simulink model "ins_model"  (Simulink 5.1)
settings: Solver=ode45  StartTime=0.0  StopTime=max(Time__s_)  RelTol=1e-3
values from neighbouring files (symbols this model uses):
  hid = [-0.2304    0.7148   -0.6309   -0.0280    0.1870    0.0308   -0.0329   -0.0106]    [meen.m]
  hir = [-0.0106   -0.0329    0.0308    0.1870   -0.0280   -0.6309    0.7148   -0.2304]    [meen.m]
  K = eye(3)    [meen.m]
  lod = [-0.0106    0.0329    0.0308  -0.1870   -0.0280    0.6309    0.7148    0.2304]    [meen.m]
  lor = [0.2304    0.7148    0.6309   -0.0280   -0.1870    0.0308    0.0329   -0.0106]    [meen.m]
  xaccel = X_Accel__g_ - mean(X_Accel__g_)    [meen.m]
  yaccel = Y_Accel__g_ - mean(Y_Accel__g_)    [meen.m]
  zaccel = Z_Accel__g_ - mean(Z_Accel__g_)    [meen.m]
undefined symbols (not defined in the file or in its folder): Customize, dspblkfdatool, Pitch__deg_, Roll__deg_, X_Accel__g_, Y_Accel__g_, Yaw_rate__deg_s_, Z_Accel__g_
libraries: dspmlti3 x12, dspsigattribs x9, simulink x3, simulink_extras x1

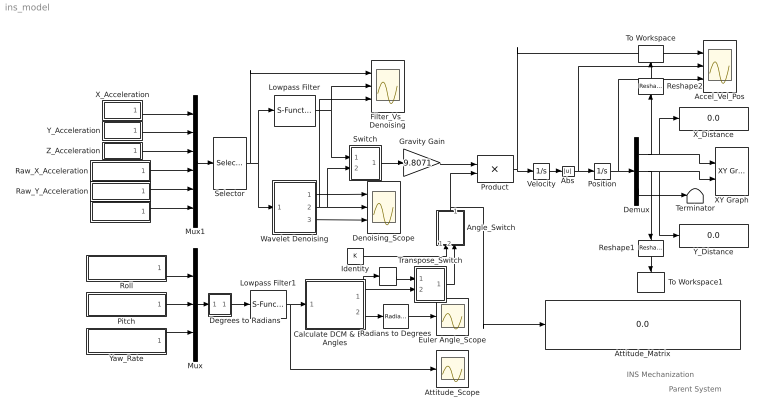
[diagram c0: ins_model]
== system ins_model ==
  note: INS Mechanization
  note: Parent System
  "    " : S-Function  FunctionName=sdspmtrnsp2  Parameters=Hermitian  mask(Transpose){Hermitian=off}
      mask help: Compute the matrix transpose. Vector input signals are treated as [Mx1] matrices. The output is always a matrix.
      mask init:
      | if(Hermitian==1),  str = 'u^H';
      | else               str = 'u^T';
      | end
  "               " : Subsystem  mask(Signal From Workspace){X=Z_Accel__g_, Ts=1/132, nsamps=1, OutputAfterFinalValue=Setting to zero}
      mask prompts: X "Signal:"; Ts "Sample time:"; nsamps "Samples per frame:"; OutputAfterFinalValue "Form output after final data value by:"
      mask help: Output signal samples obtained from the MATLAB workspace at successive sample times. A signal matrix is interpreted as having one channel per column. Signal columns may be buffered into frames by specifying a number of samples per frame greater than 1. An M x N x P signal array outputs M x N matrices at successive sample times. The samples per frame must be equal to 1 for 3 dimensional signal arrays.
      mask init:
      | [s,Ts] = dspblksfw2('init', X,Ts,nsamps);
  Abs : Abs
  Accel_Vel_Pos : Scope  NumInputPorts=3
  Angle_Switch : Subsystem  Orientation=up  mask(Manual Switch){sw=0, action=0}
      mask prompts: sw "Current setting:"
      mask help: Output toggles between two inputs by double-clicking on the block.
      mask init:
      | [x,y]=manswitch;
  Attitude_Matrix : Display
  Attitude_Scope : Scope
  Calculate DCM & Euler Angles : Subsystem
  Degrees to Radians : Subsystem
  Demux : Demux  Outputs=3
  Denoising_Scope : Scope  NumInputPorts=3
  Euler Angle_Scope : Scope
  Filter_Vs_Denoising : Scope  NumInputPorts=3
  Gravity Gain : Gain  Gain=9.8071
  Identity : Constant  Value=K
  Lowpass Filter : S-Function  StartFcn=dspblkfdatool('StartFcn');  FunctionName=sdspfilter  Parameters=1, 0, 5, 0, 1, [-0.0021051330842123276, -0.010808692912682402, -0.027404006620206183, -0.040945792508837571, -0.02656378035569611, 0.037365730644418289, 0.14346167047042629, 0.24652272003377734, 0.28957728654925807, 0.24652272003377734, 0.14346167047042629, 0.037365730644418289, -0.02656378035569611, -0.040945792508837571, -0.027404006620206183, -0.010808692912682402, -0.0021051330842123276], [1],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
  Lowpass Filter1 : S-Function  StartFcn=dspblkfdatool('StartFcn');  FunctionName=sdspfilter  Parameters=1, 0, 5, 0, 1, [-0.0021051330842123276, -0.010808692912682402, -0.027404006620206183, -0.040945792508837571, -0.02656378035569611, 0.037365730644418289, 0.14346167047042629, 0.24652272003377734, 0.28957728654925807, 0.24652272003377734, 0.14346167047042629, 0.037365730644418289, -0.02656378035569611, -0.040945792508837571, -0.027404006620206183, -0.010808692912682402, -0.0021051330842123276], [1],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
  Mux : Mux  Inputs=3
  Mux1 : Mux  Inputs=6
  Pitch : Subsystem  mask(Signal From Workspace){X=Pitch__deg_, Ts=1/132, nsamps=1, OutputAfterFinalValue=Setting to zero}
      mask prompts: X "Signal:"; Ts "Sample time:"; nsamps "Samples per frame:"; OutputAfterFinalValue "Form output after final data value by:"
      mask help: Output signal samples obtained from the MATLAB workspace at successive sample times. A signal matrix is interpreted as having one channel per column. Signal columns may be buffered into frames by specifying a number of samples per frame greater than 1. An M x N x P signal array outputs M x N matrices at successive sample times. The samples per frame must be equal to 1 for 3 dimensional signal arrays.
      mask init:
      | [s,Ts] = dspblksfw2('init', X,Ts,nsamps);
  Position : Integrator
  Product : Product  Multiplication=Matrix(*)
  Radians to Degrees : simulink_extras/Transformations/Radians to Degrees
  Raw_X_Acceleration : Subsystem  mask(Signal From Workspace){X=X_Accel__g_, Ts=1/132, nsamps=1, OutputAfterFinalValue=Setting to zero}
      mask prompts: X "Signal:"; Ts "Sample time:"; nsamps "Samples per frame:"; OutputAfterFinalValue "Form output after final data value by:"
      mask help: Output signal samples obtained from the MATLAB workspace at successive sample times. A signal matrix is interpreted as having one channel per column. Signal columns may be buffered into frames by specifying a number of samples per frame greater than 1. An M x N x P signal array outputs M x N matrices at successive sample times. The samples per frame must be equal to 1 for 3 dimensional signal arrays.
      mask init:
      | [s,Ts] = dspblksfw2('init', X,Ts,nsamps);
  Raw_Y_Acceleration : Subsystem  mask(Signal From Workspace){X=Y_Accel__g_, Ts=1/132, nsamps=1, OutputAfterFinalValue=Setting to zero}
      mask prompts: X "Signal:"; Ts "Sample time:"; nsamps "Samples per frame:"; OutputAfterFinalValue "Form output after final data value by:"
      mask help: Output signal samples obtained from the MATLAB workspace at successive sample times. A signal matrix is interpreted as having one channel per column. Signal columns may be buffered into frames by specifying a number of samples per frame greater than 1. An M x N x P signal array outputs M x N matrices at successive sample times. The samples per frame must be equal to 1 for 3 dimensional signal arrays.
      mask init:
      | [s,Ts] = dspblksfw2('init', X,Ts,nsamps);
  Reshape1 : simulink/Math Operations/Reshape  Orientation=down  OutputDimensionality=1-D array  OutputDimensions=[1,1]
  Reshape2 : simulink/Math Operations/Reshape  Orientation=up  OutputDimensionality=1-D array  OutputDimensions=[1,1]
  Roll : Subsystem  mask(Signal From Workspace){X=Roll__deg_, Ts=1/132, nsamps=1, OutputAfterFinalValue=Setting to zero}
      mask prompts: X "Signal:"; Ts "Sample time:"; nsamps "Samples per frame:"; OutputAfterFinalValue "Form output after final data value by:"
      mask help: Output signal samples obtained from the MATLAB workspace at successive sample times. A signal matrix is interpreted as having one channel per column. Signal columns may be buffered into frames by specifying a number of samples per frame greater than 1. An M x N x P signal array outputs M x N matrices at successive sample times. The samples per frame must be equal to 1 for 3 dimensional signal arrays.
      mask init:
      | [s,Ts] = dspblksfw2('init', X,Ts,nsamps);
  Selector : Selector  Elements=[1 2 3]  InputPortWidth=6
  Switch : Subsystem  mask(Manual Switch){sw=0, action=0}
      mask prompts: sw "Current setting:"
      mask help: Output toggles between two inputs by double-clicking on the block.
      mask init:
      | [x,y]=manswitch;
  Terminator : Terminator
  To Workspace : ToWorkspace  VariableName=xout  SampleTime=-1  SaveFormat=Array
  To Workspace1 : ToWorkspace  VariableName=yout  SampleTime=-1  SaveFormat=Array
  Transpose_Switch : Subsystem  mask(Manual Switch){sw=1, action=0}
      mask prompts: sw "Current setting:"
      mask help: Output toggles between two inputs by double-clicking on the block.
      mask init:
      | [x,y]=manswitch;
  Velocity : Integrator
  Wavelet Denoising : Subsystem
  XY Graph : simulink/Sinks/XY Graph  xmin=-300  xmax=300  ymin=-300  ymax=300  st=-1
  X_Acceleration : Subsystem  mask(Signal From Workspace){X=xaccel, Ts=1/132, nsamps=1, OutputAfterFinalValue=Setting to zero}
      mask prompts: X "Signal:"; Ts "Sample time:"; nsamps "Samples per frame:"; OutputAfterFinalValue "Form output after final data value by:"
      mask help: Output signal samples obtained from the MATLAB workspace at successive sample times. A signal matrix is interpreted as having one channel per column. Signal columns may be buffered into frames by specifying a number of samples per frame greater than 1. An M x N x P signal array outputs M x N matrices at successive sample times. The samples per frame must be equal to 1 for 3 dimensional signal arrays.
      mask init:
      | [s,Ts] = dspblksfw2('init', X,Ts,nsamps);
  X_Distance : Display
  Y_Acceleration : Subsystem  mask(Signal From Workspace){X=yaccel, Ts=1/132, nsamps=1, OutputAfterFinalValue=Setting to zero}
      mask prompts: X "Signal:"; Ts "Sample time:"; nsamps "Samples per frame:"; OutputAfterFinalValue "Form output after final data value by:"
      mask help: Output signal samples obtained from the MATLAB workspace at successive sample times. A signal matrix is interpreted as having one channel per column. Signal columns may be buffered into frames by specifying a number of samples per frame greater than 1. An M x N x P signal array outputs M x N matrices at successive sample times. The samples per frame must be equal to 1 for 3 dimensional signal arrays.
      mask init:
      | [s,Ts] = dspblksfw2('init', X,Ts,nsamps);
  Y_Distance : Display
  Yaw_Rate : Subsystem  mask(Signal From Workspace){X=Yaw_rate__deg_s_, Ts=1/132, nsamps=1, OutputAfterFinalValue=Setting to zero}
      mask prompts: X "Signal:"; Ts "Sample time:"; nsamps "Samples per frame:"; OutputAfterFinalValue "Form output after final data value by:"
      mask help: Output signal samples obtained from the MATLAB workspace at successive sample times. A signal matrix is interpreted as having one channel per column. Signal columns may be buffered into frames by specifying a number of samples per frame greater than 1. An M x N x P signal array outputs M x N matrices at successive sample times. The samples per frame must be equal to 1 for 3 dimensional signal arrays.
      mask init:
      | [s,Ts] = dspblksfw2('init', X,Ts,nsamps);
  Z_Acceleration : Subsystem  mask(Signal From Workspace){X=zaccel, Ts=1/132, nsamps=1, OutputAfterFinalValue=Setting to zero}
      mask prompts: X "Signal:"; Ts "Sample time:"; nsamps "Samples per frame:"; OutputAfterFinalValue "Form output after final data value by:"
      mask help: Output signal samples obtained from the MATLAB workspace at successive sample times. A signal matrix is interpreted as having one channel per column. Signal columns may be buffered into frames by specifying a number of samples per frame greater than 1. An M x N x P signal array outputs M x N matrices at successive sample times. The samples per frame must be equal to 1 for 3 dimensional signal arrays.
      mask init:
      | [s,Ts] = dspblksfw2('init', X,Ts,nsamps);
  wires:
  Mux/1 -> Degrees to Radians/1(Degrees in)
  Roll/1(Outport) -> Mux/1
  Pitch/1(Outport) -> Mux/2
  X_Acceleration/1(Outport) -> Mux1/1
  Y_Acceleration/1(Outport) -> Mux1/2
  Z_Acceleration/1(Outport) -> Mux1/3
  Mux1/1 -> Selector/1
  Calculate DCM & Euler Angles/2(Euler) -> Radians to Degrees/1
  Velocity/1 -> Abs/1
  Position/1 -> Demux/1, Accel_Vel_Pos/3
  Demux/1 -> X_Distance/1, XY Graph/1, Reshape2/1
  Demux/2 -> Y_Distance/1, XY Graph/2, Reshape1/1
  Demux/3 -> Terminator/1
  Gravity Gain/1 -> Product/1
  Product/1 -> Velocity/1, Accel_Vel_Pos/1
  Yaw_Rate/1(Outport) -> Mux/3
  Degrees to Radians/1(Radians out) -> Lowpass Filter1/1
  Switch/1(Out1) -> Gravity Gain/1
  Lowpass Filter/1 -> Switch/1(1), Filter_Vs_Denoising/2
  "               "/1(Outport) -> Mux1/6
  Raw_Y_Acceleration/1(Outport) -> Mux1/5
  Raw_X_Acceleration/1(Outport) -> Mux1/4
  Selector/1 -> Lowpass Filter/1, Wavelet Denoising/1(In1), Filter_Vs_Denoising/1
  Radians to Degrees/1 -> Euler Angle_Scope/1
  Angle_Switch/1(Out1) -> Attitude_Matrix/1, Product/2
  Identity/1 -> Angle_Switch/1(1)
  Calculate DCM & Euler Angles/1(DCM) -> Transpose_Switch/2(2), "    "/1
  "    "/1 -> Transpose_Switch/1(1)
  Lowpass Filter1/1 -> Calculate DCM & Euler Angles/1("p q r "), Attitude_Scope/1
  Transpose_Switch/1(Out1) -> Angle_Switch/2(2)
  Wavelet Denoising/2(Output) -> Switch/2(2), Denoising_Scope/2, Filter_Vs_Denoising/3
  Wavelet Denoising/1(Input) -> Denoising_Scope/1
  Wavelet Denoising/3(Residual) -> Denoising_Scope/3
  Reshape1/1 -> To Workspace1/1
  Reshape2/1 -> To Workspace/1
  Abs/1 -> Position/1, Accel_Vel_Pos/2

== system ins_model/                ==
  Frame Status : dspsigattribs/Frame Status Conversion  growRefPort=off  outframe=Sample-based
  From Workspace : FromWorkspace  VariableName=s  SampleTime=Ts  Interpolate=off  OutputAfterFinalValue=Setting to zero
  Outport : Outport  InitialOutput=0
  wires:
  From Workspace/1 -> Frame Status/1
  Frame Status/1 -> Outport/1

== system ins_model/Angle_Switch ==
  1 : Inport
  2 : Inport  Port=2
  S-Function : S-Function  FunctionName=sfun_manswitch  Parameters=boolean(0)
  Switch : Switch  Threshold=1
  Out1 : Outport
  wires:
  1/1 -> Switch/1
  2/1 -> Switch/3
  S-Function/1 -> Switch/2
  Switch/1 -> Out1/1

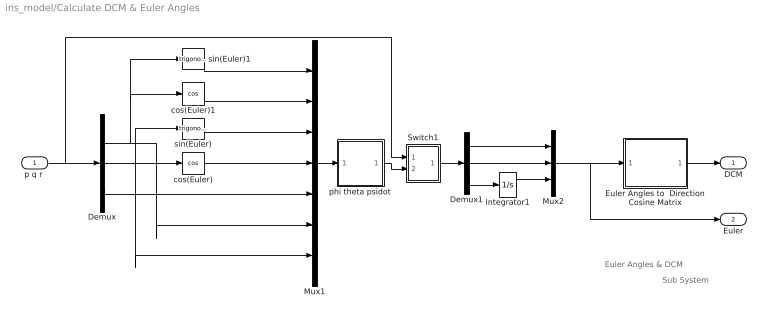
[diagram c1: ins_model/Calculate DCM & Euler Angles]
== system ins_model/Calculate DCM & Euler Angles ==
  note: Sub System
  note: Euler Angles & DCM
  "p q r " : Inport
  Demux : Demux  Outputs=3
  Demux1 : Demux  Outputs=3
  Euler Angles to  Direction Cosine Matrix : Subsystem
  Integrator1 : Integrator  ZeroCross=off
  Mux1 : Mux  Inputs=7
  Mux2 : Mux  Inputs=3
  Switch1 : Subsystem  mask(Manual Switch){sw=1, action=0}
      mask prompts: sw "Current setting:"
      mask help: Output toggles between two inputs by double-clicking on the block.
      mask init:
      | [x,y]=manswitch;
  cos(Euler) : Trigonometry  Operator=cos
  cos(Euler)1 : Trigonometry  Operator=cos
  phi theta psidot : Subsystem
  sin(Euler) : Trigonometry
  sin(Euler)1 : Trigonometry
  DCM : Outport
  Euler : Outport  Port=2
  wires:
  Euler Angles to  Direction Cosine Matrix/1(DCM) -> DCM/1
  "p q r "/1 -> Demux/1, Switch1/1(1)
  Demux/2 -> sin(Euler)/1, cos(Euler)/1, Mux1/7
  Demux/1 -> sin(Euler)1/1, cos(Euler)1/1, Mux1/6
  Demux/3 -> Mux1/5
  sin(Euler)1/1 -> Mux1/1
  cos(Euler)1/1 -> Mux1/2
  sin(Euler)/1 -> Mux1/3
  cos(Euler)/1 -> Mux1/4
  Mux1/1 -> phi theta psidot/1("           ")
  Demux1/1 -> Mux2/1
  Demux1/2 -> Mux2/2
  Demux1/3 -> Integrator1/1
  Mux2/1 -> Euler/1, Euler Angles to  Direction Cosine Matrix/1(Euler Roll Pitch Yaw)
  Integrator1/1 -> Mux2/3
  Switch1/1(Out1) -> Demux1/1
  phi theta psidot/1(phi theta psidot) -> Switch1/2(2)

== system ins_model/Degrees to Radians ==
  Degrees in : Inport
  Gain1 : Gain  Gain=pi/180
  Radians out : Outport  InitialOutput=0
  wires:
  Gain1/1 -> Radians out/1
  Degrees in/1 -> Gain1/1

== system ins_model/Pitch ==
  Frame Status : dspsigattribs/Frame Status Conversion  growRefPort=off  outframe=Sample-based
  From Workspace : FromWorkspace  VariableName=s  SampleTime=Ts  Interpolate=off  OutputAfterFinalValue=Setting to zero
  Outport : Outport  InitialOutput=0
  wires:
  Frame Status/1 -> Outport/1
  From Workspace/1 -> Frame Status/1

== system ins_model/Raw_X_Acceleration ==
  Frame Status : dspsigattribs/Frame Status Conversion  growRefPort=off  outframe=Sample-based
  From Workspace : FromWorkspace  VariableName=s  SampleTime=Ts  Interpolate=off  OutputAfterFinalValue=Setting to zero
  Outport : Outport  InitialOutput=0
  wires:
  From Workspace/1 -> Frame Status/1
  Frame Status/1 -> Outport/1

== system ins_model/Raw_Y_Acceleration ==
  Frame Status : dspsigattribs/Frame Status Conversion  growRefPort=off  outframe=Sample-based
  From Workspace : FromWorkspace  VariableName=s  SampleTime=Ts  Interpolate=off  OutputAfterFinalValue=Setting to zero
  Outport : Outport  InitialOutput=0
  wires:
  Frame Status/1 -> Outport/1
  From Workspace/1 -> Frame Status/1

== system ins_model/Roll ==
  Frame Status : dspsigattribs/Frame Status Conversion  growRefPort=off  outframe=Sample-based
  From Workspace : FromWorkspace  VariableName=s  SampleTime=Ts  Interpolate=off  OutputAfterFinalValue=Setting to zero
  Outport : Outport  InitialOutput=0
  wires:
  Frame Status/1 -> Outport/1
  From Workspace/1 -> Frame Status/1

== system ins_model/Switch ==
  1 : Inport
  2 : Inport  Port=2
  S-Function : S-Function  FunctionName=sfun_manswitch  Parameters=boolean(0)
  Switch : Switch  Threshold=1
  Out1 : Outport
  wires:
  1/1 -> Switch/1
  2/1 -> Switch/3
  S-Function/1 -> Switch/2
  Switch/1 -> Out1/1

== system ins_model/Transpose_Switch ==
  1 : Inport
  2 : Inport  Port=2
  S-Function : S-Function  FunctionName=sfun_manswitch  Parameters=boolean(1)
  Switch : Switch  Threshold=1
  Out1 : Outport
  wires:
  Switch/1 -> Out1/1
  S-Function/1 -> Switch/2
  2/1 -> Switch/3
  1/1 -> Switch/1

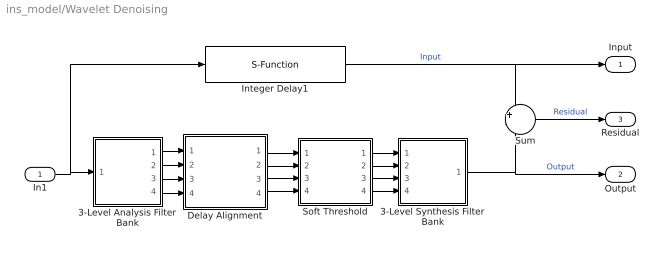
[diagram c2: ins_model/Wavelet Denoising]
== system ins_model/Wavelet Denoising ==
  In1 : Inport
  3-Level Analysis Filter Bank : Subsystem
  3-Level Synthesis Filter Bank : Subsystem
  Delay Alignment : Subsystem
  Integer Delay1 : S-Function  FunctionName=sdspdly2  Parameters=delay,ic,reset  mask(Integer Delay){delay=7*(length(lod)-1), ic=0, reset_popup=None}
      mask prompts: delay "Delay (samples):"; ic "Initial conditions:"; reset_popup "Reset port:"
      mask help: Delay discrete-time input by a fixed integer number of sample periods.
      mask init:
      | str = dspblkdly2('icon',&1,delay);
      | dx = 0.01*length(str);
      | reset = reset_popup-1;
      | if (reset == 0)
      | 	s.i1 = 1; s.i1s = '';
      | 	s.i2 = 1; s.i2s = '';
      | else
      | 	s.i1 = 1; s.i1s = 'In';
      | 	s.i2 = 2; s.i2s = 'Rst';
      | end
  Soft Threshold : Subsystem  mask(Soft Threshold){st=[3 2 1 0]}
      mask prompts: st "Vector of thresholds for each level:"
      mask help: Apply a soft threshold (deadzone transfer function) to each signal in the decomposition. First threshold applies to top-most filter bank output.
      mask init:
      | x=([-1 1 NaN 0 0 NaN -1 -.5 .5 1]+1)/2*.7+.15;
      | y=([0 0 NaN -1 1 NaN -1 0 0 1]+1)/2*.7+.05;
  Sum : Sum  Inputs=+-
  Input : Outport
  Output : Outport  Port=2
  Residual : Outport  Port=3
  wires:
  Sum/1 -> Residual/1  "Residual"
  Delay Alignment/4(Out4) -> Soft Threshold/4(in_4)
  Delay Alignment/3(Out3) -> Soft Threshold/3(in_3)
  Delay Alignment/2(Out2) -> Soft Threshold/2(in_2)
  Delay Alignment/1(Out1) -> Soft Threshold/1(in_1)
  3-Level Analysis Filter Bank/4(Out4) -> Delay Alignment/4(In4)
  3-Level Analysis Filter Bank/3(Out3) -> Delay Alignment/3(In3)
  3-Level Analysis Filter Bank/2(Out2) -> Delay Alignment/2(In2)
  3-Level Analysis Filter Bank/1(Out1) -> Delay Alignment/1(In1)
  3-Level Synthesis Filter Bank/1(Out1) -> Output/1, Sum/2  "Output"
  Integer Delay1/1 -> Input/1, Sum/1  "Input"
  Soft Threshold/4(out_4) -> 3-Level Synthesis Filter Bank/4(In4)
  Soft Threshold/3(out_3) -> 3-Level Synthesis Filter Bank/3(In3)
  Soft Threshold/2(out_2) -> 3-Level Synthesis Filter Bank/2(In2)
  Soft Threshold/1(out_1) -> 3-Level Synthesis Filter Bank/1(In1)
  In1/1 -> Integer Delay1/1, 3-Level Analysis Filter Bank/1(In1)

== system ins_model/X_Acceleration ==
  Frame Status : dspsigattribs/Frame Status Conversion  growRefPort=off  outframe=Sample-based
  From Workspace : FromWorkspace  VariableName=s  SampleTime=Ts  Interpolate=off  OutputAfterFinalValue=Setting to zero
  Outport : Outport  InitialOutput=0
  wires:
  Frame Status/1 -> Outport/1
  From Workspace/1 -> Frame Status/1

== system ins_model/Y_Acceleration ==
  Frame Status : dspsigattribs/Frame Status Conversion  growRefPort=off  outframe=Sample-based
  From Workspace : FromWorkspace  VariableName=s  SampleTime=Ts  Interpolate=off  OutputAfterFinalValue=Setting to zero
  Outport : Outport  InitialOutput=0
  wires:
  Frame Status/1 -> Outport/1
  From Workspace/1 -> Frame Status/1

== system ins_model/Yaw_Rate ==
  Frame Status : dspsigattribs/Frame Status Conversion  growRefPort=off  outframe=Sample-based
  From Workspace : FromWorkspace  VariableName=s  SampleTime=Ts  Interpolate=off  OutputAfterFinalValue=Setting to zero
  Outport : Outport  InitialOutput=0
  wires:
  Frame Status/1 -> Outport/1
  From Workspace/1 -> Frame Status/1

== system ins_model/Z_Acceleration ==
  Frame Status : dspsigattribs/Frame Status Conversion  growRefPort=off  outframe=Sample-based
  From Workspace : FromWorkspace  VariableName=s  SampleTime=Ts  Interpolate=off  OutputAfterFinalValue=Setting to zero
  Outport : Outport  InitialOutput=0
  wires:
  Frame Status/1 -> Outport/1
  From Workspace/1 -> Frame Status/1

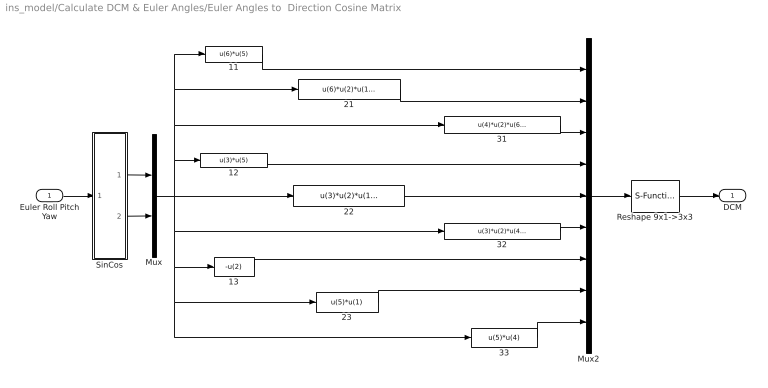
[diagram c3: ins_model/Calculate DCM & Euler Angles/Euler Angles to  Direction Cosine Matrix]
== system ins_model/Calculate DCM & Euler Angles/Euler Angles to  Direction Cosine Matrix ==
  Euler Roll Pitch Yaw : Inport
  11 : Fcn  Expr=u(6)*u(5)
  12 : Fcn  Expr=u(3)*u(5)
  13 : Fcn  Expr=-u(2)
  21 : Fcn  Expr=u(6)*u(2)*u(1)-u(3)*u(4)
  22 : Fcn  Expr=u(3)*u(2)*u(1)+u(6)*u(4)
  23 : Fcn  Expr=u(5)*u(1)
  31 : Fcn  Expr=u(4)*u(2)*u(6)+u(3)*u(1)
  32 : Fcn  Expr=u(3)*u(2)*u(4)-u(6)*u(1)
  33 : Fcn  Expr=u(5)*u(4)
  Mux : Mux  Inputs=2
  Mux2 : Mux  Inputs=9
  Reshape 9x1->3x3 : S-Function  FunctionName=sreshape  Parameters=OutputDimensionality, OutputDimensions  mask(Reshape){OutputDimensionality=Customize, OutputDimensions=[3,3]}
      mask prompts: OutputDimensionality "Output dimensionality:"; OutputDimensions "Output dimensions:"
      mask help: Change the dimensions of a vector or matrix input signal. Output - a one-dimensional array (vector), - a column vector (Mx1 matrix), - a row vector (1xN matrix), or - a matrix or vector with specified dimensions, e.g., [M, N] or [W].
      mask init:
      | s = reshapemask(gcbh,'init');
  SinCos : Subsystem
  DCM : Outport  InitialOutput=0
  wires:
  33/1 -> Mux2/9
  23/1 -> Mux2/8
  13/1 -> Mux2/7
  32/1 -> Mux2/6
  22/1 -> Mux2/5
  12/1 -> Mux2/4
  31/1 -> Mux2/3
  21/1 -> Mux2/2
  11/1 -> Mux2/1
  Mux2/1 -> Reshape 9x1->3x3/1
  Reshape 9x1->3x3/1 -> DCM/1
  SinCos/1(sin(theta)) -> Mux/1
  SinCos/2(cos(theta)) -> Mux/2
  Euler Roll Pitch Yaw/1 -> SinCos/1(theta)
  Mux/1 -> 22/1, 11/1, 21/1, 31/1, 12/1, 32/1, 13/1, 23/1, 33/1

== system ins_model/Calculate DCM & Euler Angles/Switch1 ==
  1 : Inport
  2 : Inport  Port=2
  S-Function : S-Function  FunctionName=sfun_manswitch  Parameters=boolean(1)
  Switch : Switch  Threshold=1
  Out1 : Outport
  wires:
  1/1 -> Switch/1
  2/1 -> Switch/3
  S-Function/1 -> Switch/2
  Switch/1 -> Out1/1

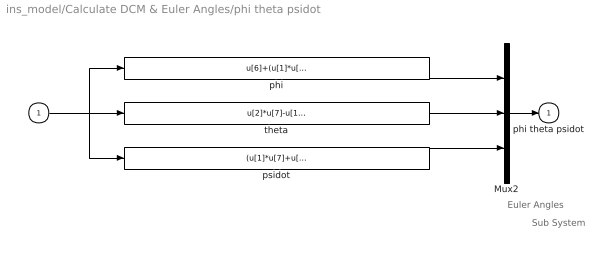
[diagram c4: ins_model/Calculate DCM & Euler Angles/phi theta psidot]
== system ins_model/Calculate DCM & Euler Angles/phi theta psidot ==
  note: Euler Angles
  note: Sub System
  "           " : Inport
  Mux2 : Mux  Inputs=3
  phi : Fcn  Expr=u[6]+(u[1]*u[7]+u[2]*u[5])*(u[3]/u[4])
  psidot : Fcn  Expr=(u[1]*u[7]+u[2]*u[5])/u[4]
  theta : Fcn  Expr=u[2]*u[7]-u[1]*u[5]
  phi theta psidot : Outport  InitialOutput=0
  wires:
  phi/1 -> Mux2/1
  theta/1 -> Mux2/2
  psidot/1 -> Mux2/3
  "           "/1 -> theta/1, phi/1, psidot/1
  Mux2/1 -> phi theta psidot/1

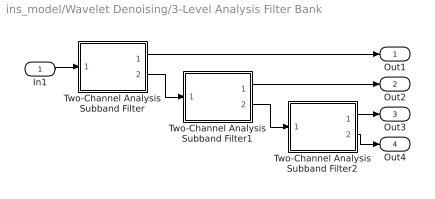
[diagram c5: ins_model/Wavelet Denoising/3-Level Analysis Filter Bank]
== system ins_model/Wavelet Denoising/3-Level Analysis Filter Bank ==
  In1 : Inport
  Two-Channel Analysis Subband Filter : Subsystem  mask(Two-Channel Analysis Subband Filter){lpf=lod, hpf=hid, framing=Maintain input frame size}
      mask prompts: lpf "Lowpass FIR filter coefficients:"; hpf "Highpass FIR filter coefficients:"
      mask help: Decomposes a signal into a high-frequency subband (Hi band) and a low-frequency subband (Lo band) using the specified highpass and lowpass FIR filters. Each subband has half the bandwidth and half the sample rate of the original signal. Usually, the highpass and lowpass filters should be half-band filters designed to complement each other. This block accepts sample- and frame-based inputs of all sizes. To implement a multi-level filter bank that decomposes a signal into more than two subbands, use the Dyadic Analysis Filter Bank in the Multirate Filters library (accepts only frame-based inputs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
      mask init:
      | dspblk2chabank('init');
  Two-Channel Analysis Subband Filter1 : Subsystem  mask(Two-Channel Analysis Subband Filter){lpf=lod, hpf=hid, framing=Maintain input frame size}
      mask prompts: lpf "Lowpass FIR filter coefficients:"; hpf "Highpass FIR filter coefficients:"
      mask help: Decomposes a signal into a high-frequency subband (Hi band) and a low-frequency subband (Lo band) using the specified highpass and lowpass FIR filters. Each subband has half the bandwidth and half the sample rate of the original signal. Usually, the highpass and lowpass filters should be half-band filters designed to complement each other. This block accepts sample- and frame-based inputs of all sizes. To implement a multi-level filter bank that decomposes a signal into more than two subbands, use the Dyadic Analysis Filter Bank in the Multirate Filters library (accepts only frame-based inputs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
      mask init:
      | dspblk2chabank('init');
  Two-Channel Analysis Subband Filter2 : Subsystem  mask(Two-Channel Analysis Subband Filter){lpf=lod, hpf=hid, framing=Maintain input frame size}
      mask prompts: lpf "Lowpass FIR filter coefficients:"; hpf "Highpass FIR filter coefficients:"
      mask help: Decomposes a signal into a high-frequency subband (Hi band) and a low-frequency subband (Lo band) using the specified highpass and lowpass FIR filters. Each subband has half the bandwidth and half the sample rate of the original signal. Usually, the highpass and lowpass filters should be half-band filters designed to complement each other. This block accepts sample- and frame-based inputs of all sizes. To implement a multi-level filter bank that decomposes a signal into more than two subbands, use the Dyadic Analysis Filter Bank in the Multirate Filters library (accepts only frame-based inputs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
      mask init:
      | dspblk2chabank('init');
  Out1 : Outport
  Out2 : Outport  Port=2
  Out3 : Outport  Port=3
  Out4 : Outport  Port=4
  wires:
  Two-Channel Analysis Subband Filter/2(Out2) -> Two-Channel Analysis Subband Filter1/1(in)
  Two-Channel Analysis Subband Filter1/2(Out2) -> Two-Channel Analysis Subband Filter2/1(in)
  Two-Channel Analysis Subband Filter/1(out1) -> Out1/1
  In1/1 -> Two-Channel Analysis Subband Filter/1(in)
  Two-Channel Analysis Subband Filter1/1(out1) -> Out2/1
  Two-Channel Analysis Subband Filter2/1(out1) -> Out3/1
  Two-Channel Analysis Subband Filter2/2(Out2) -> Out4/1

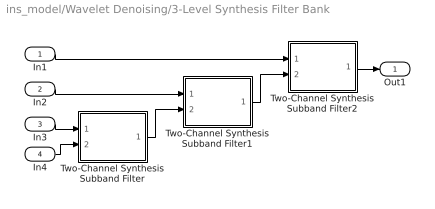
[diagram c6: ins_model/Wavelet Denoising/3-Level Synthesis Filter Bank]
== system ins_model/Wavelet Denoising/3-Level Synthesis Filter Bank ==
  In1 : Inport
  In2 : Inport  Port=2
  In3 : Inport  Port=3
  In4 : Inport  Port=4
  Two-Channel Synthesis Subband Filter : Subsystem  mask(Two-Channel Synthesis Subband Filter){lpf=lor, hpf=hir, framing=Maintain input frame size}
      mask prompts: lpf "Lowpass FIR filter coefficients:"; hpf "Highpass FIR filter coefficients:"
      mask help: Reconstructs a signal from a high-frequency subband (Hi band) and a low-frequnecy subband (Lo band) using the specified highpass and lowpass FIR filters. The input subbands should have the same bandwidths and sample rates. Usually, the highpass and lowpass filters should be half-band filters designed to complement each other. This block accepts sample- and frame-based inputs of all sizes. To create a multi-level filter bank that reconstructs a signal from more than two subbands, use the Dyadic Synthesis Filter Bank in the Multirate Filters library (has more constraints on its inputs).
      mask init:
      | dspblk2chsbank('init');
  Two-Channel Synthesis Subband Filter1 : Subsystem  mask(Two-Channel Synthesis Subband Filter){lpf=lor, hpf=hir, framing=Maintain input frame size}
      mask prompts: lpf "Lowpass FIR filter coefficients:"; hpf "Highpass FIR filter coefficients:"
      mask help: Reconstructs a signal from a high-frequency subband (Hi band) and a low-frequnecy subband (Lo band) using the specified highpass and lowpass FIR filters. The input subbands should have the same bandwidths and sample rates. Usually, the highpass and lowpass filters should be half-band filters designed to complement each other. This block accepts sample- and frame-based inputs of all sizes. To create a multi-level filter bank that reconstructs a signal from more than two subbands, use the Dyadic Synthesis Filter Bank in the Multirate Filters library (has more constraints on its inputs).
      mask init:
      | dspblk2chsbank('init');
  Two-Channel Synthesis Subband Filter2 : Subsystem  mask(Two-Channel Synthesis Subband Filter){lpf=lor, hpf=hir, framing=Maintain input frame size}
      mask prompts: lpf "Lowpass FIR filter coefficients:"; hpf "Highpass FIR filter coefficients:"
      mask help: Reconstructs a signal from a high-frequency subband (Hi band) and a low-frequnecy subband (Lo band) using the specified highpass and lowpass FIR filters. The input subbands should have the same bandwidths and sample rates. Usually, the highpass and lowpass filters should be half-band filters designed to complement each other. This block accepts sample- and frame-based inputs of all sizes. To create a multi-level filter bank that reconstructs a signal from more than two subbands, use the Dyadic Synthesis Filter Bank in the Multirate Filters library (has more constraints on its inputs).
      mask init:
      | dspblk2chsbank('init');
  Out1 : Outport
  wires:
  Two-Channel Synthesis Subband Filter/1(Out1) -> Two-Channel Synthesis Subband Filter1/2(In2)
  Two-Channel Synthesis Subband Filter1/1(Out1) -> Two-Channel Synthesis Subband Filter2/2(In2)
  In1/1 -> Two-Channel Synthesis Subband Filter2/1(In1)
  Two-Channel Synthesis Subband Filter2/1(Out1) -> Out1/1
  In2/1 -> Two-Channel Synthesis Subband Filter1/1(In1)
  In3/1 -> Two-Channel Synthesis Subband Filter/1(In1)
  In4/1 -> Two-Channel Synthesis Subband Filter/2(In2)

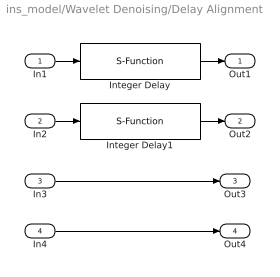
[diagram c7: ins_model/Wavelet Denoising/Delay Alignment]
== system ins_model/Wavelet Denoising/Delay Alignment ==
  In1 : Inport
  In2 : Inport  Port=2
  In3 : Inport  Port=3
  In4 : Inport  Port=4
  Integer Delay : S-Function  FunctionName=sdspdly2  Parameters=delay,ic,reset  mask(Integer Delay){delay=3*(length(lod)-1), ic=0, reset_popup=None}
      mask prompts: delay "Delay (samples):"; ic "Initial conditions:"; reset_popup "Reset port:"
      mask help: Delay discrete-time input by a fixed integer number of sample periods.
      mask init:
      | str = dspblkdly2('icon',&1,delay);
      | dx = 0.01*length(str);
      | reset = reset_popup-1;
      | if (reset == 0)
      | 	s.i1 = 1; s.i1s = '';
      | 	s.i2 = 1; s.i2s = '';
      | else
      | 	s.i1 = 1; s.i1s = 'In';
      | 	s.i2 = 2; s.i2s = 'Rst';
      | end
  Integer Delay1 : S-Function  FunctionName=sdspdly2  Parameters=delay,ic,reset  mask(Integer Delay){delay=length(lod) - 1, ic=0, reset_popup=None}
      mask prompts: delay "Delay (samples):"; ic "Initial conditions:"; reset_popup "Reset port:"
      mask help: Delay discrete-time input by a fixed integer number of sample periods.
      mask init:
      | str = dspblkdly2('icon',&1,delay);
      | dx = 0.01*length(str);
      | reset = reset_popup-1;
      | if (reset == 0)
      | 	s.i1 = 1; s.i1s = '';
      | 	s.i2 = 1; s.i2s = '';
      | else
      | 	s.i1 = 1; s.i1s = 'In';
      | 	s.i2 = 2; s.i2s = 'Rst';
      | end
  Out1 : Outport
  Out2 : Outport  Port=2
  Out3 : Outport  Port=3
  Out4 : Outport  Port=4
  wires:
  Integer Delay/1 -> Out1/1
  In1/1 -> Integer Delay/1
  Integer Delay1/1 -> Out2/1
  In2/1 -> Integer Delay1/1
  In4/1 -> Out4/1
  In3/1 -> Out3/1

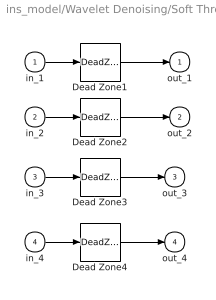
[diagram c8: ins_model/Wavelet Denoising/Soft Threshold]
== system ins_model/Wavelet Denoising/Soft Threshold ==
  in_1 : Inport
  in_2 : Inport  Port=2
  in_3 : Inport  Port=3
  in_4 : Inport  Port=4
  Dead Zone1 : DeadZone  LowerValue=-st(1)  UpperValue=st(1)  ZeroCross=off
  Dead Zone2 : DeadZone  LowerValue=-st(2)  UpperValue=st(2)  ZeroCross=off
  Dead Zone3 : DeadZone  LowerValue=-st(3)  UpperValue=st(3)  ZeroCross=off
  Dead Zone4 : DeadZone  LowerValue=-st(4)  UpperValue=st(4)  ZeroCross=off
  out_1 : Outport  InitialOutput=0
  out_2 : Outport  Port=2  InitialOutput=0
  out_3 : Outport  Port=3  InitialOutput=0
  out_4 : Outport  Port=4  InitialOutput=0
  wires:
  Dead Zone4/1 -> out_4/1
  in_4/1 -> Dead Zone4/1
  Dead Zone3/1 -> out_3/1
  in_3/1 -> Dead Zone3/1
  Dead Zone2/1 -> out_2/1
  in_2/1 -> Dead Zone2/1
  Dead Zone1/1 -> out_1/1
  in_1/1 -> Dead Zone1/1

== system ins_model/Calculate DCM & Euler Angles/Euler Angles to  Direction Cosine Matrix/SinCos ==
  theta : Inport
  cosine : Trigonometry  Operator=cos
  sine : Trigonometry
  sin(theta) : Outport
  cos(theta) : Outport  Port=2
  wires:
  cosine/1 -> cos(theta)/1
  sine/1 -> sin(theta)/1
  theta/1 -> cosine/1, sine/1

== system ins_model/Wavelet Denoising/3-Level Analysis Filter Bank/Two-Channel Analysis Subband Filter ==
  in : Inport
  FIR Decimation : dspmlti3/FIR Decimation  h=hid  D=2  framing=Maintain input frame size  outputBufInitCond=0  roundingMode=Floor  overflowMode=off
  FIR Decimation1 : dspmlti3/FIR Decimation  h=lod  D=2  framing=Maintain input frame size  outputBufInitCond=0  roundingMode=Floor  overflowMode=off
  out1 : Outport
  Out2 : Outport  Port=2
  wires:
  FIR Decimation1/1 -> Out2/1
  in/1 -> FIR Decimation1/1, FIR Decimation/1
  FIR Decimation/1 -> out1/1

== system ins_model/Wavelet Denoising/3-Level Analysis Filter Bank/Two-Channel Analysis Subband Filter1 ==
  in : Inport
  FIR Decimation : dspmlti3/FIR Decimation  h=hid  D=2  framing=Maintain input frame size  outputBufInitCond=0  roundingMode=Floor  overflowMode=off
  FIR Decimation1 : dspmlti3/FIR Decimation  h=lod  D=2  framing=Maintain input frame size  outputBufInitCond=0  roundingMode=Floor  overflowMode=off
  out1 : Outport
  Out2 : Outport  Port=2
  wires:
  FIR Decimation1/1 -> Out2/1
  in/1 -> FIR Decimation1/1, FIR Decimation/1
  FIR Decimation/1 -> out1/1

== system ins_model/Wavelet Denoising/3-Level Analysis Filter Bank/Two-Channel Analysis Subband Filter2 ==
  in : Inport
  FIR Decimation : dspmlti3/FIR Decimation  h=hid  D=2  framing=Maintain input frame size  outputBufInitCond=0  roundingMode=Floor  overflowMode=off
  FIR Decimation1 : dspmlti3/FIR Decimation  h=lod  D=2  framing=Maintain input frame size  outputBufInitCond=0  roundingMode=Floor  overflowMode=off
  out1 : Outport
  Out2 : Outport  Port=2
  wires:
  FIR Decimation1/1 -> Out2/1
  in/1 -> FIR Decimation1/1, FIR Decimation/1
  FIR Decimation/1 -> out1/1

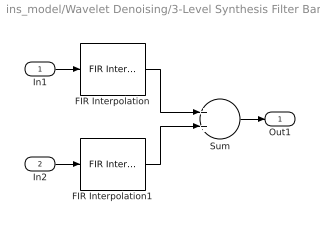
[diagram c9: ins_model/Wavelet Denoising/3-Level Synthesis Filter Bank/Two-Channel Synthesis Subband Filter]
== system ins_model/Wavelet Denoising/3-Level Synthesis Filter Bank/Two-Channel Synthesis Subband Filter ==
  In1 : Inport
  In2 : Inport  Port=2
  FIR Interpolation : dspmlti3/FIR Interpolation  h=hir  L=2  framing=Maintain input frame size  outputBufInitCond=0  roundingMode=Floor  overflowMode=off
  FIR Interpolation1 : dspmlti3/FIR Interpolation  h=lor  L=2  framing=Maintain input frame size  outputBufInitCond=0  roundingMode=Floor  overflowMode=off
  Sum : Sum
  Out1 : Outport
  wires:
  FIR Interpolation/1 -> Sum/1
  FIR Interpolation1/1 -> Sum/2
  In1/1 -> FIR Interpolation/1
  Sum/1 -> Out1/1
  In2/1 -> FIR Interpolation1/1

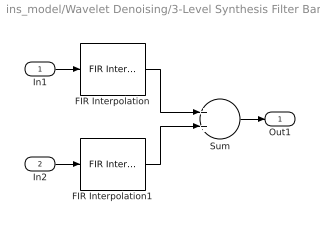
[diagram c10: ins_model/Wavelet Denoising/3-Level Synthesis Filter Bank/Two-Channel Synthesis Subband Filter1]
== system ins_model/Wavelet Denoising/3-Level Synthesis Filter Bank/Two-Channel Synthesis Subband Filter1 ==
  In1 : Inport
  In2 : Inport  Port=2
  FIR Interpolation : dspmlti3/FIR Interpolation  h=hir  L=2  framing=Maintain input frame size  outputBufInitCond=0  roundingMode=Floor  overflowMode=off
  FIR Interpolation1 : dspmlti3/FIR Interpolation  h=lor  L=2  framing=Maintain input frame size  outputBufInitCond=0  roundingMode=Floor  overflowMode=off
  Sum : Sum
  Out1 : Outport
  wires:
  FIR Interpolation/1 -> Sum/1
  FIR Interpolation1/1 -> Sum/2
  In1/1 -> FIR Interpolation/1
  Sum/1 -> Out1/1
  In2/1 -> FIR Interpolation1/1

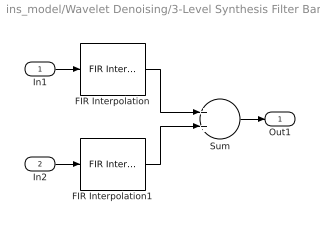
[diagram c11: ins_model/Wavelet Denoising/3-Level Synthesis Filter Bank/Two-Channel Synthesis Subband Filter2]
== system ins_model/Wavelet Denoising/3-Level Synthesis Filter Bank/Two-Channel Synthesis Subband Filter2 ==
  In1 : Inport
  In2 : Inport  Port=2
  FIR Interpolation : dspmlti3/FIR Interpolation  h=hir  L=2  framing=Maintain input frame size  outputBufInitCond=0  roundingMode=Floor  overflowMode=off
  FIR Interpolation1 : dspmlti3/FIR Interpolation  h=lor  L=2  framing=Maintain input frame size  outputBufInitCond=0  roundingMode=Floor  overflowMode=off
  Sum : Sum
  Out1 : Outport
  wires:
  FIR Interpolation/1 -> Sum/1
  FIR Interpolation1/1 -> Sum/2
  In1/1 -> FIR Interpolation/1
  Sum/1 -> Out1/1
  In2/1 -> FIR Interpolation1/1
